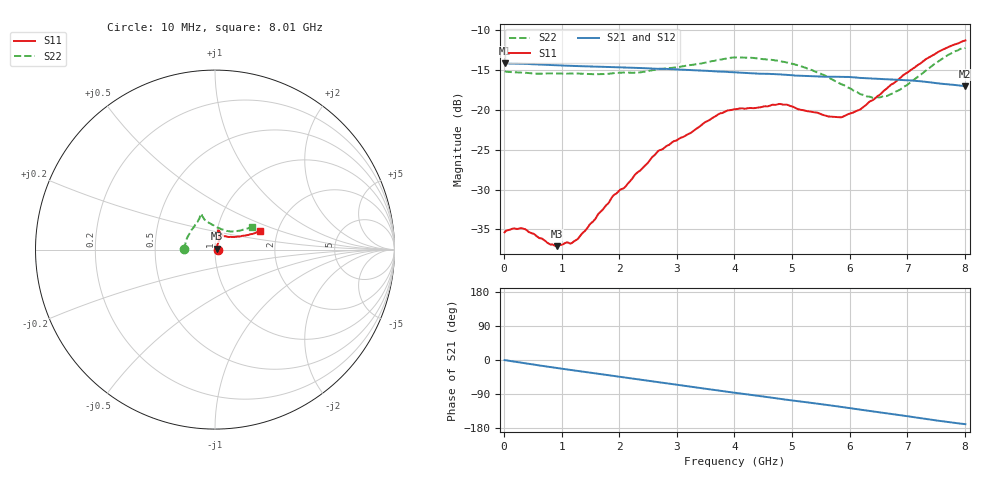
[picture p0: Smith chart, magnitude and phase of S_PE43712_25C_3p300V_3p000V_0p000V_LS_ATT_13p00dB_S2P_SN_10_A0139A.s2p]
! DEVICE ID: PE43712
! File Path: z:\PE43713\PE43713_CHAR_NOM_04292014\AMB\3p300\LS_ATT_13p00dB\PE43713_AMB_3p300V_3p000V_0p000V_LS_ATT_13p00dB_S2P_SN_10_A0139A.s2p
! Serial: 10
! Lot: A0139A
! Temp: 25C
! VDD: 3.300
! VSS: 0.000
! Control_Hi: 3.000
! Control_Lo: 0.000
! Attenuation Step: 13.00dB
! Port 1: RF1
! Port 2: RF2
! ThroughPath:1-2
! IDD: 0.0001471663
! ISS: -2.068e-007
#  Hz  S  RI  R  50
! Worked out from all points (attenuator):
!   801 points, 10 MHz to 8.01 GHz, reference 50 ohm
!   highest |S21| = -14.18 dB at 10 MHz (marker M1); lowest = -17.1 dB at 8 GHz (marker M2)
!   lowest |S11| = -37.1 dB at 920 MHz (marker M3), VSWR 1.03, Z = 51.3 + j0.554 ohm
!   |S11| at or under -10 dB: start of sweep to end of sweep
!   |S22| runs from -18.5 to -12.2 dB; largest |S21 - S12| = 0.0007
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1e7  0.0171 0.000294  0.1954 -0.00101  0.1955 -0.000982  -0.1738 0.00111
3.3e8  0.018 0.000319  0.1919 -0.0268  0.1917 -0.0266  -0.1694 0.0193
9.2e8  0.0129 0.0054  0.1772 -0.0686  0.1773 -0.0687  -0.161 0.0504
1.18e9  0.011 0.00963  0.1682 -0.0846  0.1682 -0.0847  -0.1561 0.0642
1.35e9  0.0112 0.0124  0.1619 -0.0946  0.1619 -0.0947  -0.1519 0.0719
1.9e9  0.0134 0.0258  0.1375 -0.1236  0.1375 -0.1236  -0.1353 0.1021
2.11e9  0.0145 0.0297  0.1269 -0.1332  0.1268 -0.1332  -0.1297 0.1112
2.68e9  0.0228 0.0504  0.0945 -0.1538  0.0944 -0.1538  -0.1055 0.146
3.72e9  0.0234 0.0906  0.0289 -0.1713  0.0287 -0.1713  -0.0832 0.1873
4.01e9  0.022 0.0984  0.0106 -0.1713  0.0105 -0.1713  -0.0833 0.1957
4.79e9  0.0198 0.1069  -0.0356 -0.1626  -0.0357 -0.1628  -0.0725 0.1886
5.35e9  0.0302 0.092  -0.0648 -0.1488  -0.0648 -0.1487  -0.0582 0.1671
5.64e9  0.0404 0.0812  -0.0785 -0.1407  -0.0784 -0.1408  -0.0399 0.1535
5.88e9  0.0511 0.0745  -0.0907 -0.1327  -0.0905 -0.1327  -0.0207 0.1422
6.17e9  0.0701 0.0711  -0.1034 -0.12  -0.1032 -0.1202  0.00773 0.1259
6.38e9  0.0887 0.0715  -0.1108 -0.111  -0.1106 -0.1109  0.031 0.1154
6.68e9  0.12 0.0716  -0.1209 -0.0968  -0.1207 -0.0969  0.067 0.1038
7e9  0.1527 0.0764  -0.1302 -0.0803  -0.13 -0.0803  0.1015 0.1008
7.36e9  0.1934 0.0848  -0.1365 -0.0596  -0.1364 -0.0596  0.1443 0.1076
7.72e9  0.2291 0.0946  -0.1384 -0.0402  -0.1384 -0.0403  0.1864 0.1198
8e9  0.2497 0.1052  -0.1379 -0.0264  -0.1377 -0.0266  0.2075 0.1276
8.01e9  0.2503 0.1059  -0.138 -0.0261  -0.1377 -0.0263  0.2081 0.1278
